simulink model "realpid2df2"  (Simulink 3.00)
settings: Solver=ode45  SolverMode=SingleTasking  StartTime=0.0  StopTime=10  FixedStep=st_size  MaxStep=st_size  RelTol=1e-5  AbsTol=1e-6
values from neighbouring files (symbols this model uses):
  d_through_p = get(MAIN_MENU(19),'Value')    [cback.m]    (also in imcmenu.m = 0)
  Disturb = Setpoint    [mimo_MSF1DF_sim.m]    (also in mimo_MSF2DF_sim.m)
  K = 1/kpd    [imc2pseucon.m]    (also in imc2pseudo.m)
  Satlb = temp1    [cback.m]    (also in imcmenu.m = str2num(satlbs))
  Satub = temp1    [cback.m]    (also in imcmenu.m = str2num(satubs))
  Setpoint = zeros(1,n)    [mimo_MSF1DF_sim.m]    (also in mimo_MSF2DF_sim.m)
undefined symbols (not defined in the file or in its folder): denPd, numPd, pdeadx, Pre_fil_den, Pre_fil_num, TauD, TauI, XdenPs, XnumPs

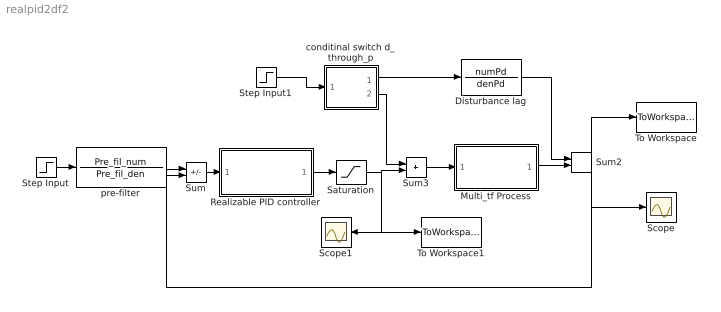
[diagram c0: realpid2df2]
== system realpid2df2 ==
  Disturbance lag : TransferFcn  Numerator=numPd  Denominator=denPd
  Multi_tf Process : Subsystem
  Realizable PID controller : Subsystem
  Saturation : Saturate  UpperLimit=Satub  LowerLimit=Satlb
  Scope : Scope
  Scope1 : Scope
  Step Input : Step  Time=0  Before=0  After=Setpoint  SampleTime=0
  Step Input1 : Step  Time=0  Before=0  After=Disturb  SampleTime=0
  Sum : Sum  Inputs=+-  SaturateOnIntegerOverflow=on
  Sum2 : Sum  Inputs=++  SaturateOnIntegerOverflow=on
  Sum3 : Sum  Inputs=++  SaturateOnIntegerOverflow=on
  To Workspace : ToWorkspace  VariableName=simout  SampleTime=-1  SaveFormat=Matrix
  To Workspace1 : ToWorkspace  VariableName=effort  SampleTime=-1  SaveFormat=Matrix
  conditinal switch d_through_p : Subsystem  Description=pass input signal through out1 if condition is true.
  pre-filter : TransferFcn  Numerator=Pre_fil_num  Denominator=Pre_fil_den
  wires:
  Step Input/1 -> pre-filter/1
  pre-filter/1 -> Sum/1
  Sum/1 -> Realizable PID controller/1(In1)
  Realizable PID controller/1(Out1) -> Saturation/1
  Sum3/1 -> Multi_tf Process/1(In1)
  Multi_tf Process/1(Out1) -> Sum2/2
  conditinal switch d_through_p/2(Out1) -> Sum3/1
  conditinal switch d_through_p/1(Out2) -> Disturbance lag/1
  Step Input1/1 -> conditinal switch d_through_p/1(In)
  Saturation/1 -> Sum3/2, To Workspace1/1, Scope1/1
  Disturbance lag/1 -> Sum2/1
  Sum2/1 -> Sum/2, To Workspace/1, Scope/1

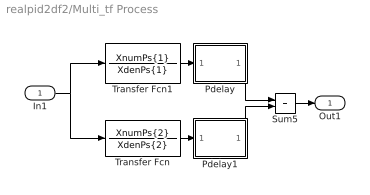
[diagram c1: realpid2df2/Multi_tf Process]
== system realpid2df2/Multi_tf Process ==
  In1 : Inport  Port=1  PortWidth=-1  SampleTime=-1  DataType=auto
  Pdelay : Subsystem
  Pdelay1 : Subsystem
  Sum5 : Sum  Inputs=++  SaturateOnIntegerOverflow=on
  Transfer Fcn : TransferFcn  Numerator=XnumPs{2}  Denominator=XdenPs{2}
  Transfer Fcn1 : TransferFcn  Numerator=XnumPs{1}  Denominator=XdenPs{1}
  Out1 : Outport  Port=1  InitialOutput=0
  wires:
  Transfer Fcn1/1 -> Pdelay/1(In1)
  Transfer Fcn/1 -> Pdelay1/1(In1)
  In1/1 -> Transfer Fcn1/1, Transfer Fcn/1
  Sum5/1 -> Out1/1
  Pdelay/1(Out1) -> Sum5/1
  Pdelay1/1(Out1) -> Sum5/2

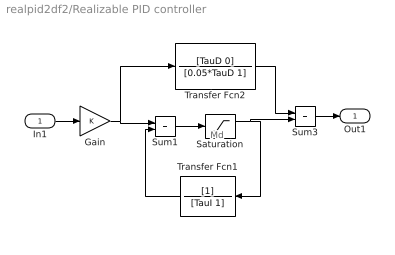
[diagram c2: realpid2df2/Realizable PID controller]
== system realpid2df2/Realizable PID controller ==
  note: Md
  In1 : Inport  Port=1  PortWidth=-1  SampleTime=-1  DataType=auto
  Gain : Gain  Gain=K  SaturateOnIntegerOverflow=on
  Saturation : Saturate  UpperLimit=Satub  LowerLimit=Satlb
  Sum1 : Sum  Inputs=++  SaturateOnIntegerOverflow=on
  Sum3 : Sum  Inputs=++  SaturateOnIntegerOverflow=on
  Transfer Fcn1 : TransferFcn  Orientation=left  Numerator=[1]  Denominator=[TauI 1]
  Transfer Fcn2 : TransferFcn  Numerator=[TauD 0]  Denominator=[0.05*TauD 1]
  Out1 : Outport  Port=1  InitialOutput=0
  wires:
  Sum1/1 -> Saturation/1
  Transfer Fcn1/1 -> Sum1/2
  Gain/1 -> Sum1/1, Transfer Fcn2/1
  Saturation/1 -> Transfer Fcn1/1, Sum3/2
  Transfer Fcn2/1 -> Sum3/1
  Sum3/1 -> Out1/1
  In1/1 -> Gain/1

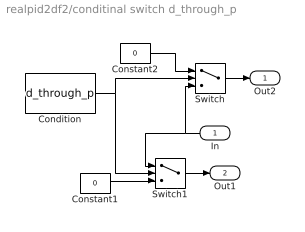
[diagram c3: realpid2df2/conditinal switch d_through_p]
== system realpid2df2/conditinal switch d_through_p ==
  In : Inport  Orientation=left  Port=1  PortWidth=-1  SampleTime=-1  DataType=auto
  Condition : Constant  Value=d_through_p
  Constant1 : Constant  Value=0
  Constant2 : Constant  Value=0
  Switch : Switch  Threshold=1
  Switch1 : Switch  Threshold=1
  Out2 : Outport  Port=1  InitialOutput=0
  Out1 : Outport  Port=2  InitialOutput=0
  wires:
  In/1 -> Switch/3, Switch1/1
  Condition/1 -> Switch1/2, Switch/2
  Constant1/1 -> Switch1/3
  Constant2/1 -> Switch/1
  Switch/1 -> Out2/1
  Switch1/1 -> Out1/1

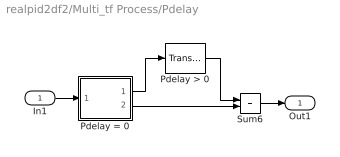
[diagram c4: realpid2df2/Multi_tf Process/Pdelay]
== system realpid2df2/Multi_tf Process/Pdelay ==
  In1 : Inport  Port=1  PortWidth=-1  SampleTime=-1  DataType=auto
  Pdelay > 0 : TransportDelay  DelayTime=pdeadx(1)  InitialInput=0  BufferSize=1024
  Pdelay = 0 : Subsystem  Description=pass input signal through out1 if condition is true.
  Sum6 : Sum  Inputs=++  SaturateOnIntegerOverflow=on
  Out1 : Outport  Port=1
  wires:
  Pdelay = 0/1(Out2) -> Pdelay > 0/1
  Pdelay > 0/1 -> Sum6/1
  Pdelay = 0/2(Out1) -> Sum6/2
  In1/1 -> Pdelay = 0/1(In)
  Sum6/1 -> Out1/1

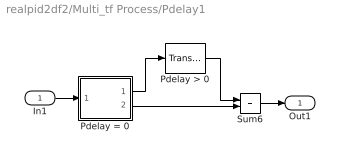
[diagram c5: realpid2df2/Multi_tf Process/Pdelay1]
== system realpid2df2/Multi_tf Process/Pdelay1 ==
  In1 : Inport  Port=1  PortWidth=-1  SampleTime=-1  DataType=auto
  Pdelay > 0 : TransportDelay  DelayTime=pdeadx(2)  InitialInput=0  BufferSize=1024
  Pdelay = 0 : Subsystem  Description=pass input signal through out1 if condition is true.
  Sum6 : Sum  Inputs=++  SaturateOnIntegerOverflow=on
  Out1 : Outport  Port=1
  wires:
  Pdelay = 0/1(Out2) -> Pdelay > 0/1
  Pdelay > 0/1 -> Sum6/1
  Pdelay = 0/2(Out1) -> Sum6/2
  In1/1 -> Pdelay = 0/1(In)
  Sum6/1 -> Out1/1

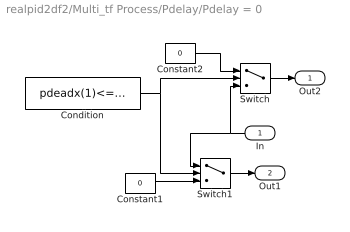
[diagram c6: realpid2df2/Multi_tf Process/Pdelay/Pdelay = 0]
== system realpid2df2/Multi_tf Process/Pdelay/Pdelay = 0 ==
  In : Inport  Orientation=left  Port=1  PortWidth=-1  SampleTime=-1  DataType=auto
  Condition : Constant  Value=pdeadx(1)<=3*eps
  Constant1 : Constant  Value=0
  Constant2 : Constant  Value=0
  Switch : Switch  Threshold=1
  Switch1 : Switch  Threshold=1
  Out2 : Outport  Port=1  InitialOutput=0
  Out1 : Outport  Port=2  InitialOutput=0
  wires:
  In/1 -> Switch/3, Switch1/1
  Condition/1 -> Switch1/2, Switch/2
  Constant1/1 -> Switch1/3
  Constant2/1 -> Switch/1
  Switch/1 -> Out2/1
  Switch1/1 -> Out1/1

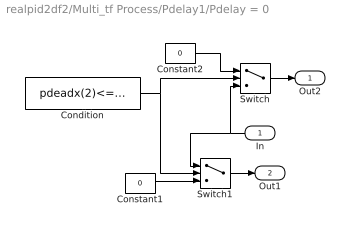
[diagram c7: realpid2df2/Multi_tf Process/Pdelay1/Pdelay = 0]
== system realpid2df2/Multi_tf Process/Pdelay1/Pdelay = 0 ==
  In : Inport  Orientation=left  Port=1  PortWidth=-1  SampleTime=-1  DataType=auto
  Condition : Constant  Value=pdeadx(2)<=3*eps
  Constant1 : Constant  Value=0
  Constant2 : Constant  Value=0
  Switch : Switch  Threshold=1
  Switch1 : Switch  Threshold=1
  Out2 : Outport  Port=1  InitialOutput=0
  Out1 : Outport  Port=2  InitialOutput=0
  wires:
  In/1 -> Switch/3, Switch1/1
  Condition/1 -> Switch1/2, Switch/2
  Constant1/1 -> Switch1/3
  Constant2/1 -> Switch/1
  Switch/1 -> Out2/1
  Switch1/1 -> Out1/1
